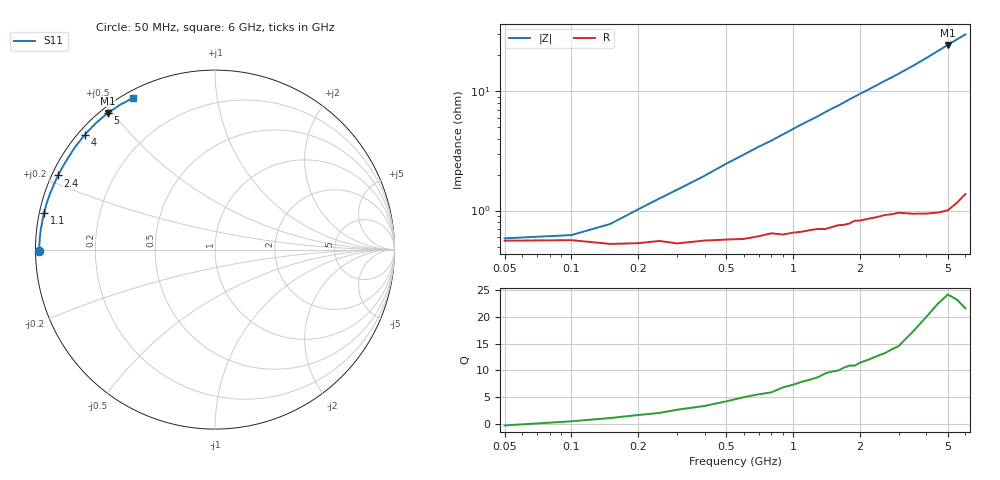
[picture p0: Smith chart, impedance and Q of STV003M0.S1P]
! SIEMENS Discrete & RF Semiconductors
! BA892
! Si PIN Diode in SCD-80
! IF = 3 mA
! S-Parameters:  September  1997
# GHz  S  MA  R  50
!  f  S11
! GHz  MAG  ANG
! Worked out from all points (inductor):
!   34 points, 50 MHz to 6 GHz, reference 50 ohm
!   read as one part to ground: L = 765 pH near 400 MHz
!   highest Q = 23.2 at 5 GHz (marker M1), where L = 774 pH
!   S11 on the Smith chart (normalised r, x): 50 MHz: 0.01, -0.00; 1.1 GHz: 0.01, +0.11; 2.4 GHz: 0.02, +0.22; 4 GHz: 0.02, +0.38; 5 GHz: 0.02, +0.49; 6 GHz: 0.03, +0.59
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0.05  0.9779 -179.6
0.1  0.9776 179.4
0.15  0.9792 178.7
0.2  0.9789 178.0
0.25  0.978 177.4
0.3  0.979 176.8
0.4  0.9778 175.7
0.5  0.9774 174.5
0.6  0.9772 173.4
0.7  0.976 172.3
0.8  0.9747 171.3
0.9  0.9753 170.2
1.1  0.974 168.0
1.3  0.9727 166.0
1.4  0.9728 164.9
1.5  0.9718 163.8
1.6  0.9709 162.9
1.8  0.9701 160.7
2.2  0.9677 156.7
2.4  0.9669 154.7
2.6  0.9659 152.7
2.8  0.9657 150.8
3.5  0.9666 143.8
4  0.9675 138.6
4.5  0.9681 133.3
5  0.968 128.1
5.5  0.9646 123.1
6  0.9602 118.5
